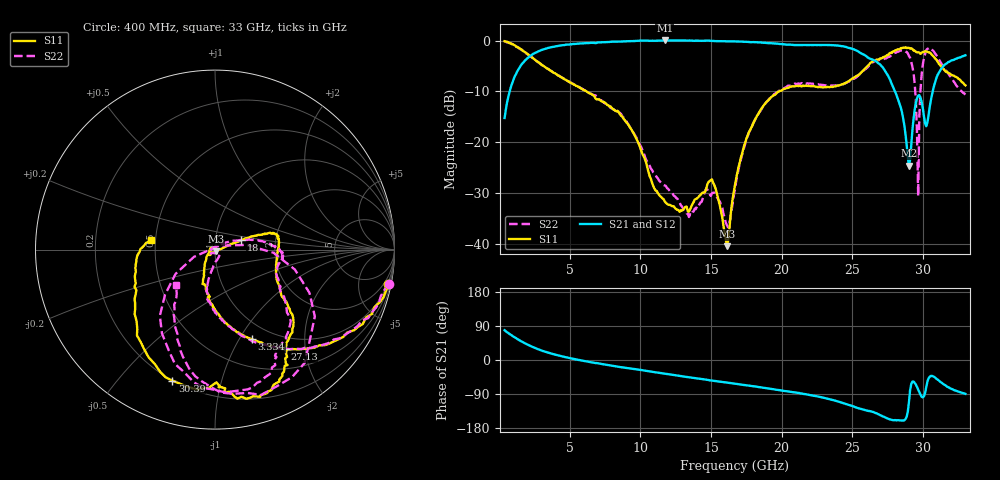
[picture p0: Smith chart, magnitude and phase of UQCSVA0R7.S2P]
!  Part Number  UQCSVA0R7  Mounting Orientation: Horizontal
!  Description: Ultra Low ESR Microwave capacitors
!  Application: Coupling, Bypass, Tuning, DC Block
!  Filters, Matching
# GHZ S DB R 50
! Freq  |S11|  S11 Ph  |S21|  S21 Ph  |S12|  S12 Ph  |S22|  S22 Ph
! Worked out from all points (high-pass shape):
!   401 points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, 400 MHz to 33 GHz, reference 50 ohm
!   highest |S21| = 0.02 dB at 11.73 GHz (marker M1); lowest = -24.6 dB at 29.01 GHz (marker M2)
!   |S21| within 3 dB of the highest: 2.241 GHz to 25.93 GHz (23.69 GHz wide, 168 % of centre); 32.919 GHz to end of sweep
!   lowest |S11| = -40.4 dB at 16.13 GHz (marker M3), VSWR 1.02, Z = 50.4 - j0.866 ohm
!   |S11| at or under -10 dB: 6.2 GHz to 19.82 GHz (13.62 GHz wide, 105 % of centre)
!   |S22| runs from -36.7 to -0.1 dB; largest |S21 - S12| = 0.0087
!   S11 on the Smith chart (normalised r, x): 400 MHz: 1, -10; 3.334 GHz: 0.80, -1.13; 18 GHz: 1.34, +0.14; 27.13 GHz: 0.79, -1.62; 30.39 GHz: 0.20, -0.71; 33 GHz: 0.47, +0.06
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0.4  -0.13 -11.4  -15.22 78.5  -15.23 78.4  -0.11 -11.0
1.46  -1.56 -37.9  -5.32 51.8  -5.30 52.1  -1.61 -37.0
3.334  -5.35 -67.7  -1.57 21.1  -1.56 21.1  -5.37 -68.7
5.861  -9.51 -90.0  -0.58 -1.4  -0.58 -1.5  -9.44 -91.4
9.039  -16.16 -112.9  -0.14 -21.0  -0.16 -21.2  -15.99 -102.1
11.321  -30.29 -171.5  -0.01 -33.6  -0.03 -33.8  -27.49 -57.5
11.729  -31.61 162.6  0.02 -36.0  0.01 -36.1  -28.50 -44.5
13.44  -33.64 -179.8  0.01 -45.6  -0.01 -45.7  -34.68 -92.4
15.07  -27.27 -137.7  -0.08 -54.5  -0.08 -54.4  -30.00 -151.0
16.13  -40.41 -64.3  -0.16 -59.7  -0.16 -59.7  -36.30 138.4
16.7  -28.37 9.1  -0.16 -62.6  -0.18 -62.5  -29.17 48.2
18.004  -16.17 19.3  -0.30 -69.1  -0.31 -69.3  -16.18 19.9
22.161  -8.98 3.8  -0.89 -93.3  -0.88 -93.3  -8.46 -7.6
27.132  -3.39 -55.1  -5.20 -148.5  -5.25 -148.2  -3.69 -57.6
27.621  -2.54 -58.1  -7.41 -156.3  -7.43 -156.1  -3.19 -60.8
29.007  -1.42 -78.1  -24.61 -110.6  -24.39 -109.6  -3.04 -104.0
29.333  -1.98 -83.9  -15.41 -56.9  -15.36 -58.0  -6.37 -129.8
29.659  -2.31 -88.5  -10.84 -78.3  -10.91 -78.4  -30.55 45.4
30.066  -2.24 -94.6  -14.83 -95.8  -14.79 -95.0  -3.49 -33.8
30.392  -2.30 -108.0  -14.73 -48.9  -14.63 -48.9  -1.56 -65.4
31.126  -4.58 -137.8  -6.33 -54.3  -6.34 -54.8  -3.69 -104.1
33  -8.80 171.6  -2.89 -89.4  -2.88 -89.6  -10.63 -138.1
